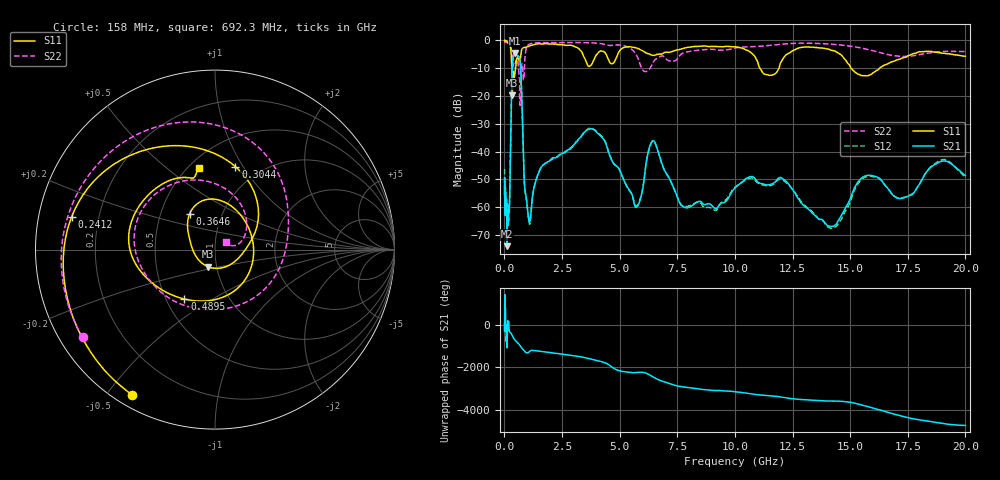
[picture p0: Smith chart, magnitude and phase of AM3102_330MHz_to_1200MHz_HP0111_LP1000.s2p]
! Date/Time: Tue, Sep 11, 2018 5:16 PM
! Network Analyzer: Agilent Technologies E8362B Rev: A.07.50.63
! Sweep from 0.010 to 20.000 GHz, 1601 Points, Sweep Type: LOG
! Power Supply: 4.949 V, 0.001 A
# Hz S DB R 50
!freq MagS11 AngS11 MagS21 AngS21 MagS12 AngS12 MagS22 AngS22
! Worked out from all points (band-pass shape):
!   1601 points, 10 MHz to 20 GHz, reference 50 ohm
!   highest |S21| = -4.54 dB at 471.2 MHz (marker M1); lowest = -74.0 dB at 109.1 MHz (marker M2)
!   |S21| within 3 dB of the highest: 359.4 MHz to 681.6 MHz (322.2 MHz wide, 61.9 % of centre)
!   lowest |S11| = -19.7 dB at 341.1 MHz (marker M3), VSWR 1.23, Z = 45.4 - j8.7 ohm
!   |S11| at or under -10 dB: 317.4 MHz to 486.9 MHz (169.4 MHz wide, 42.1 % of centre); 11.09 GHz to 11.91 GHz (825.7 MHz wide, 7.18 % of centre); 15.04 GHz to 16.28 GHz (1.238 GHz wide, 7.91 % of centre)
!   |S22| runs from -23.4 to -0.3 dB; largest |S21 - S12| = 0.011
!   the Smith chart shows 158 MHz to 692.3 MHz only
!   S11 on the Smith chart (normalised r, x): 158 MHz: 0.05, -0.58; 241.2 MHz: 0.10, +0.11; 304.4 MHz: 0.77, +0.93; 364.6 MHz: 0.70, +0.30; 489.5 MHz: 0.62, -0.38; 692.3 MHz: 0.56, +0.65
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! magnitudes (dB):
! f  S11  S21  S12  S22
! 10 MHz  0.0  -54.0  -46.2  -0.3
! 35.55 MHz  0.0  -61.8  -59.2  -0.5
! 109.1 MHz  -0.3  -74.0  -62.3  -0.8
! 126.4 MHz  -0.4  -61.2  -64.9  -0.9
! 158 MHz  -0.6  -65.6  -64.7  -1.1
! 241.2 MHz  -1.7  -52.1  -51.1  -1.8
! 304.4 MHz  -6.4  -21.1  -21.2  -3.5
! 341.1 MHz  -19.7  -9.8  -9.9  -6.7
! 364.6 MHz  -12.2  -7.1  -7.2  -8.3
! 447.2 MHz  -12.5  -4.6  -4.6  -8.9
! 471.2 MHz  -11.1  -4.5  -4.6  -8.2
! 489.5 MHz  -9.8  -4.6  -4.7  -7.7
! 692.3 MHz  -6.6  -8.5  -8.5  -22.4
! 1.067 GHz  -2.0  -64.7  -65.1  -1.4
! 1.59 GHz  -1.3  -45.7  -45.8  -0.8
! 3.793 GHz  -8.6  -31.8  -31.6  -0.8
! 5.652 GHz  -2.5  -59.3  -59.0  -4.3
! 6.457 GHz  -5.4  -36.0  -36.2  -7.8
! 7.808 GHz  -2.8  -59.9  -59.7  -4.4
! 11.92 GHz  -9.9  -49.4  -49.9  -1.5
! 14.07 GHz  -3.1  -66.7  -67.2  -1.3
! 20 GHz  -5.7  -48.6  -49.3  -4.0
